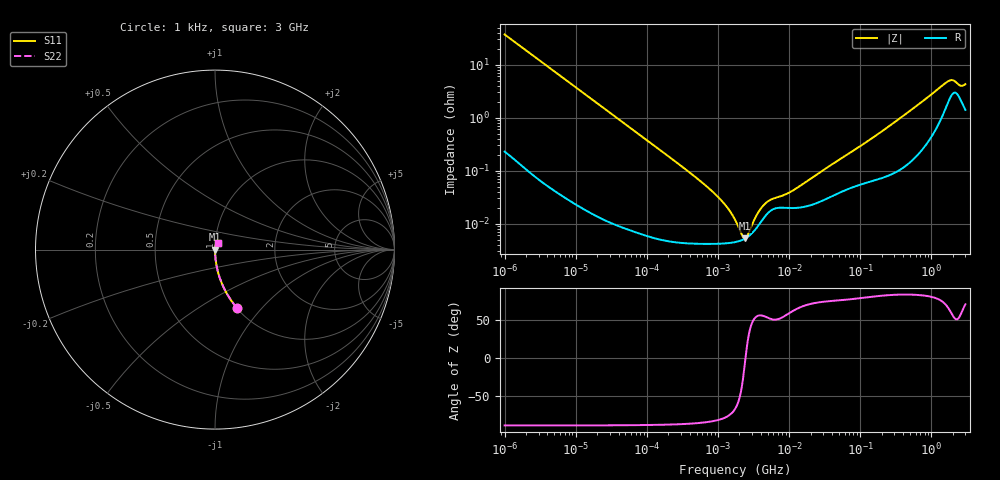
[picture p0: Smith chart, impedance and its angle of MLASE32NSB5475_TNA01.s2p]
! MLASE32NSB5475_TNA01  S-PARAMETER MODEL  ( Standard Model )
! Model Generated by TAIYO YUDEN Corporation (http://www.ty-top.com)
! Version 1.0
! TAIYO YUDEN Control No. 220601
! Copyright(c) 2009 TAIYO YUDEN CO.,LTD. All Rights Reserved.
! Product Description (link to TY-COMPAS)
! https://ds.yuden.co.jp/TYCOMPAS/or/detail?pn=MLASE32NSB5475KTNA01&u=M
! Products Name : Multilayer Ceramic Capacitors
! Characteristics :
!  Capacitance : 4.7 [uF] , Rated Voltage : 16 [V] , TCC : B / X5R
!  Case Size : 3.2 x 2.5 / 0.126 x 0.098 [mm/inch] , Thickness : 1.9 / 0.075 [mm/inch]
!  (Conditions: Temperature = 25 [degC] , DC Bias Voltage = 0 [V])
! External Node Assignments :
!  1  o---| |---o  2
! GND o---------o GND
! Frequency Range : 1kHz  -  3GHz  [ 401 STEP ]
# MHZ S RI R 50
! Freq[MHz].  S11 Real  S11 Imag  S21 Real  S21 Imag  S12 Real  S12 Imag  S22 Real  S22 Imag
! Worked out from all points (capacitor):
!   401 points, 1 kHz to 3 GHz, reference 50 ohm
!   read as one part in series: C = 4.28 uF near 1.077 kHz
!   lowest |Z| = 5.29 mohm at 2.423 MHz (marker M1)
!   series resonance near 2.435 MHz, so ESL is about 1 nH
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0.001  0.1224 -0.3247  0.8776 0.3247  0.8776 0.3247  0.1224 -0.3247
0.001685  0.0475 -0.2098  0.9525 0.2098  0.9525 0.2098  0.0475 -0.2098
0.00306  0.0152 -0.1198  0.9848 0.1198  0.9848 0.1198  0.0152 -0.1198
0.01216  0.00114 -0.0307  0.9989 0.0307  0.9989 0.0307  0.00114 -0.0307
0.147855  5.72e-05 -0.00254  0.9999 0.00254  0.9999 0.00254  5.72e-05 -0.00254
0.452501  4.27e-05 -0.000808  1 0.000808  1 0.000808  4.27e-05 -0.000808
0.852899  4.18e-05 -0.000392  1 0.000392  1 0.000392  4.18e-05 -0.000392
1.285341  4.27e-05 -0.000216  1 0.000216  1 0.000216  4.27e-05 -0.000216
1.732051  4.5e-05 -0.000111  1 0.000111  1 0.000111  4.5e-05 -0.000111
1.937042  4.67e-05 -7.42e-05  1 7.42e-05  1 7.42e-05  4.67e-05 -7.42e-05
2.422679  5.29e-05 -1.68e-06  0.9999 1.68e-06  0.9999 1.68e-06  5.29e-05 -1.68e-06
2.812335  6.1e-05 4.73e-05  0.9999 -4.73e-05  0.9999 -4.73e-05  6.1e-05 4.73e-05
3.03007  6.7e-05 7.21e-05  0.9999 -7.21e-05  0.9999 -7.21e-05  6.7e-05 7.21e-05
4.083148  0.000112 0.000167  0.9999 -0.000167  0.9999 -0.000167  0.000112 0.000167
5.106836  0.000162 0.000214  0.9998 -0.000214  0.9998 -0.000214  0.000162 0.000214
9.991309  0.000198 0.000332  0.9998 -0.000332  0.9998 -0.000332  0.000198 0.000332
21.06097  0.000229 0.000704  0.9998 -0.000704  0.9998 -0.000704  0.000229 0.000704
256.0921  0.000867 0.00691  0.9991 -0.00691  0.9991 -0.00691  0.000867 0.00691
1714.862  0.0209 0.0429  0.9791 -0.0429  0.9791 -0.0429  0.0209 0.0429
1990.675  0.0292 0.04  0.9708 -0.04  0.9708 -0.04  0.0292 0.04
2584.342  0.0219 0.0325  0.9781 -0.0325  0.9781 -0.0325  0.0219 0.0325
3000  0.0154 0.0394  0.9846 -0.0394  0.9846 -0.0394  0.0154 0.0394
